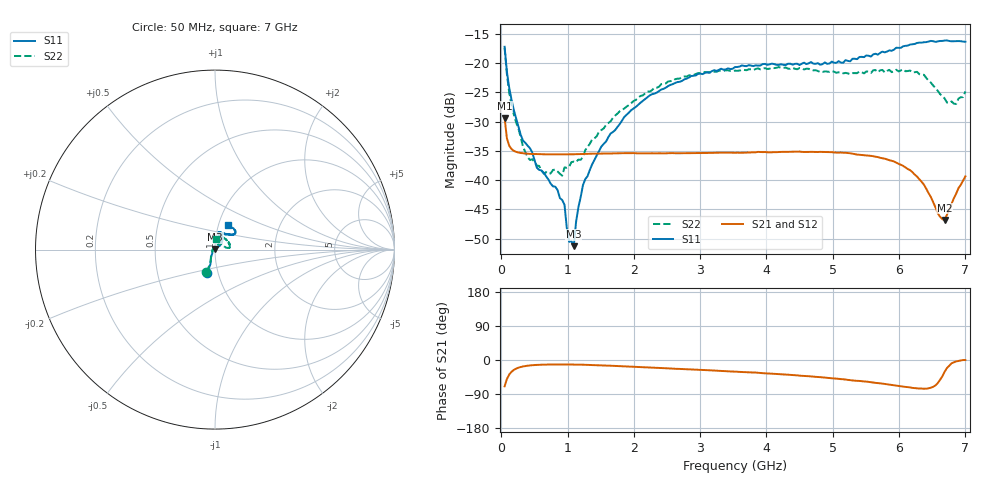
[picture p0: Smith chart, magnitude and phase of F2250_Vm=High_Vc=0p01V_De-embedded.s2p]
! Integrated Device Technology
! Corporate Headquarters
! 6024 Silver Creek Valley Road
! San Jose, CA 95138  USA
! Phone:  1-408-284-8200
! Toll Free:  1-800-223-1366
! Webpage:  http://www.idt.com/
! Timing and RF Division
! 515 Groton Road, Suite 102
! Westford, MA 01886-6024
! Device:  F2250
! Description: Voltage Variable RF Attenuator
! Frequency:  50.0 -  6000.00 MHz
! Package:  3x3 mm Thin QFN Plastic Package: 16 pin
! Ports:  2 RF, 3 DC
!  Pin  1  = GND
!  Pin  2  = NC
!  Pin  3  = RF1  = Port 1
!  Pin  4  = NC
!  Pin  5  = GND
!  Pin  6  = GND
!  Pin  7  = GND
!  Pin  8  = GND
!  Pin  9  = NC
!  Pin 10  = RF2  = Port 2
!  Pin 11  = NC
!  Pin 12  = GND
!  Pin 13  = GND
!  Pin 14  = VCNTRL
!  Pin 15  = VDD
!  Pin 16  = VMODE
! Vcntrl:  0.010 Volts
! Vmode:  +3.300 Volts
! Vdd:  +3.30  Volts
! Current:  1.242 mA
! Data:  The device was measured on a the F2250 evaluation board which has
!  individual transmission lines to the RF pins.  Data was collected
!  using a calibrated network analyzer.  The evaluation board was
!  de-embedded using a TRL calibration technique.
!  The reference plane is the edge of the package pin.
! Misc:  SN 10
!  Action Tracker AT0258
! Date Measured:  2014-11-26
! Date:  2015-10-15  MJV
! Note:
!  Integrated Device Technology supplies this data as a sample of measured
!  data at the package pin for this product.  Your particular data for this
!  product may vary.
!  Data was taken at 25 degrees C.
!  Integrated Device Technology reserves the right to change this data at anytime.
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# GHz S dB R 50
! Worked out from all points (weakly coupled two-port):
!   201 points, 50 MHz to 7 GHz, reference 50 ohm
!   highest |S21| = -29.38 dB at 50 MHz (marker M1); lowest = -46.8 dB at 6.687 GHz (marker M2)
!   lowest |S11| = -51.3 dB at 1.093 GHz (marker M3), VSWR 1.01, Z = 50 + j0.272 ohm
!   |S11| at or under -10 dB: start of sweep to end of sweep
!   |S22| runs from -39.2 to -17.4 dB; largest |S21 - S12| = 5.2e-05
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0.05  -17.18 -108.5  -29.38 -69.5  -29.38 -69.5  -17.37 -110.6
0.08475  -21.47 -107.4  -32.86 -50.1  -32.86 -50.1  -21.87 -109.0
0.15425  -26.22 -116.5  -34.68 -31.0  -34.68 -31.0  -27.10 -120.7
0.29325  -32.26 -127.4  -35.35 -18.5  -35.35 -18.4  -32.66 -133.5
0.3975  -34.11 -142.2  -35.48 -15.1  -35.48 -15.0  -36.07 -158.3
0.5365  -37.87 -154.7  -35.55 -13.0  -35.55 -12.9  -37.50 -180.0
0.64075  -38.75 -162.6  -35.58 -12.2  -35.58 -12.2  -38.89 160.7
0.91875  -43.40 155.9  -35.60 -11.8  -35.60 -11.8  -39.23 127.9
0.9535  -44.21 171.1  -35.60 -11.8  -35.60 -11.8  -37.82 124.2
1.023  -50.57 140.0  -35.59 -11.9  -35.59 -11.9  -37.71 108.0
1.0925  -51.30 90.1  -35.57 -12.0  -35.58 -12.0  -36.82 98.9
1.12725  -47.20 61.9  -35.56 -12.1  -35.56 -12.1  -36.92 91.8
1.2315  -40.86 41.1  -35.53 -12.5  -35.52 -12.5  -36.04 77.2
1.6485  -32.03 41.2  -35.44 -15.2  -35.44 -15.2  -29.92 60.0
2.37825  -24.75 46.7  -35.39 -21.0  -35.40 -21.0  -24.02 53.9
3.525  -20.65 71.7  -35.32 -30.6  -35.32 -30.6  -21.26 73.0
4.7065  -20.07 72.0  -35.15 -43.9  -35.15 -43.9  -21.21 70.4
5.85325  -17.79 40.5  -36.58 -64.9  -36.58 -64.9  -21.13 23.4
6.27025  -16.52 39.4  -39.39 -74.5  -39.40 -74.5  -21.46 8.6
6.68725  -16.11 47.9  -46.81 -31.0  -46.81 -30.7  -26.03 28.4
6.861  -16.21 54.5  -42.31 -3.7  -42.27 -3.8  -26.95 57.4
7  -16.32 62.4  -39.35 -0.1  -39.32 -0.3  -24.82 83.6
